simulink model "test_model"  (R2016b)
settings: Solver=VariableStepAuto  StartTime=0.0  StopTime=runtime  RelTol=1e-3
InitFcn:
  | clear mex
  | delete test_model_sfun.mexw64
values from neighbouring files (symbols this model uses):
  delta_T = 4 * [ 0,  0,  2.351e-4 ]    [modelParameters.m]
  Delta_T = cell(1,4)    [modelParameters.m]
  F_D = 1*randn(3,1)    [modelParameters.m]
  g = 9.81    [modelParameters.m]    (also in analyzeIMU_data.m = 9.8; getMomentOfInertia.m = 9.80665)
  Gamma_H = cell(1,4)    [modelParameters.m]
  have_motor_transient = 1    [modelParameters.m]
  height_controlled_o = (((Rm*If        + (((omega0_o * 2 * Rm * Kv * Kq      * Kd + 1)^2) - 1)/(4* Rm*Kv^2*Kq      * Kd))/Vb)*(Pmax - Pmin) + Pmin)    [modelParameters.m]
  i_0 = cell(1,4)    [modelParameters.m]
  If = 0.3836    [modelParameters.m]    (also in thrustDragConstantCalculations.m = [If0; If1; If2; If3]; Kd_error.m = I_0 * sign(rotor_speed_0) + I_1 * rotor_speed_0 + I_2 * roto)
  J = diag([ 0.0130 0.0140 0.0285 ])    [modelParameters.m]    (also in J_calc_bifilar.m = (16*pi^2*L./(m*g.*D.^2))\(t./n).^2)
  J_L = m_L/12*diag([y_L^2+z_L^2,x_L^2+z_L^2,x_L^2+y_L^2])    [modelParameters.m]
  J_r = cell(1,4)    [modelParameters.m]
  Jreq = 4.2012e-05    [modelParameters.m]
  Jxx = 0.0130    (= 0.013)    [modelParameters.m]
  Jyy = 0.0140    (= 0.014)    [modelParameters.m]
  Jzz = 0.0285    [modelParameters.m]
  K_d = cell(1,4)    [modelParameters.m]
  K_E = cell(1,4)    [modelParameters.m]
  K_H = cell(1,4)    [modelParameters.m]
  K_Q = cell(1,4)    [modelParameters.m]
  K_T = cell(1,4)    [modelParameters.m]
  K_V = cell(1,4)    [modelParameters.m]
  Kd = 1.4852e-07    [modelParameters.m]    (also in calcDragConstant.m = ((A'*A)^-1)*A'*b; thrustDragConstantCalculations.m = calcDragConstant(data, Pmin, Pmax, Rm, Kv, Kq, If); Kd_error.m = 1.0317e-07)
  Kh = 3.4574e-04    (= 0.00034574)    [modelParameters.m]
  Ki_mahony = 0.001    [modelParameters.m]
  Kp_mahony = 0.4    [modelParameters.m]
  Kq = 96.3422    [modelParameters.m]    (also in thrustDragConstantCalculations.m; Kd_error.m)
  Kt = 1.2007e-05    [modelParameters.m]    (also in calcThrustConstant.m = ((A'*A)^(-1))*(A'*T); thrustDragConstantCalculations.m = calcThrustConstant(data))
  Kv = 96.3422    [modelParameters.m]    (also in thrustDragConstantCalculations.m; Kd_error.m)
  m = 1.216    [modelParameters.m]
  m_L = 0    [modelParameters.m]
  omega0_o = sqrt((m*g)/(4*Kt))    [modelParameters.m]
  omega1_o = sqrt((m*g)/(4*Kt))    [modelParameters.m]
  omega2_o = sqrt((m*g)/(4*Kt))    [modelParameters.m]
  omega3_o = sqrt((m*g)/(4*Kt))    [modelParameters.m]
  omega_0 = cell(1,4)    [modelParameters.m]
  p0 = 0    [modelParameters.m]
  p_0 = cell(1,4)    [modelParameters.m]
  p_max = cell(1,4)    [modelParameters.m]
  phi0 = 0    [modelParameters.m]
  pitch_o = 0    [modelParameters.m]
  pitchrate_o = 0    [modelParameters.m]
  Pmax = 1    [modelParameters.m]    (also in thrustDragConstantCalculations.m = 200000; Kd_error.m = 200000)
  Pmin = 0    [modelParameters.m]    (also in thrustDragConstantCalculations.m = 100000; Kd_error.m = 100000)
  psi0 = 0    [modelParameters.m]
  q0 = 0    [modelParameters.m]
  Q_D = 0.05*randn(3,1)    [modelParameters.m]
  r0 = 0    [modelParameters.m]
  R_m = cell(1,4)    [modelParameters.m]
  r_oc = [ 0 ; 0 ; 0 ]    [modelParameters.m]
  r_oL = [0; 0; 0]    [modelParameters.m]
  rhx = 0.16    [modelParameters.m]
  rhy = 0.16    [modelParameters.m]
  rhz = 0.03    [modelParameters.m]
  Rm = 0.235    [modelParameters.m]    (also in thrustDragConstantCalculations.m = 0.2308; Kd_error.m = 0.2308)
  roll_o = 0    [modelParameters.m]
  rollrate_o = 0    [modelParameters.m]
  Tc = 0.04    [modelParameters.m]
  theta0 = 0    [modelParameters.m]
  Tq = 0.005    [modelParameters.m]
  u0 = 0    [modelParameters.m]
  v0 = 0    [modelParameters.m]
  Vb = 12.3    [modelParameters.m]    (also in calcDragConstant.m = [data.(6); data.(6); data.(6); data.(6)]; Kd_error.m = data.(6))
  w0 = 0    [modelParameters.m]
  x0 = 0    [modelParameters.m]
  x_controlled_o = 0    [modelParameters.m]
  x_o = 0    [modelParameters.m]
  x_vel_o = 0    [modelParameters.m]
  y0 = 0    [modelParameters.m]
  y_controlled_o = 0    [modelParameters.m]
  y_o = 0    [modelParameters.m]
  y_vel_o = 0    [modelParameters.m]
  yaw_controlled_o = 0    [modelParameters.m]
  yaw_o = 0    [modelParameters.m]
  yawrate_o = 0    [modelParameters.m]
  z0 = 0    [modelParameters.m]
  z_o = 0    [modelParameters.m]
  z_vel_o = 0    [modelParameters.m]
undefined symbols (not defined in the file or in its folder): Gamma_Omega, Gamma_T, Ki, Kp, r_h, slope, start, Ts, X0
libraries: simulink x32, Derivative x26, dsparch4 x6, vrlib x4
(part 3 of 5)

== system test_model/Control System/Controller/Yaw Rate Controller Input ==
  note: 1) Add Subsystem or Model blocks as valid variant choices. 2) You cannot connect blocks at this level. At simulation, connectivity is automatically determined, based on the active variant and port name matching.
  yawrate_error_model : Inport
  yawrate_model : Inport  Port=2
  Feedback : Subsystem  VariantControl=logAnalysisToggle==0
  yawrate error : Subsystem  VariantControl=logAnalysisToggle==1
  yawrate_error : Outport
  yawrate : Outport  Port=2

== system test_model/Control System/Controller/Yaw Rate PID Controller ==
  yawrate_error : Inport
  yawrate : Inport  Port=2
  Add : Sum  Inputs=+-
  Discrete D Controller : Derivative/Discrete D Controller  Kd=Kd  a=a
  Discrete PI Controller : simulink/Continuous/PID Controller  Controller=PI  TimeDomain=Discrete-time  SampleTime=Ts  IntegratorMethod=Forward Euler  FilterMethod=Forward Euler  Form=Parallel  UseFilter=on  ControllerParametersSource=internal  P=Kp  I=Ki  D=0  N=100  InitialConditionSource=internal  InitialConditionForIntegrator=0  InitialConditionForFilter=0  ExternalReset=none  LimitOutput=off  UpperSaturationLimit=inf  LowerSaturationLimit=-inf  LinearizeAsGain=off  AntiWindupMode=none  Kb=1  TrackingMode=off  Kt=1  PParamMin=[]  PParamMax=[]  IParamMin=[]  IParamMax=[]  DParamMin=[]  DParamMax=[]  NParamMin=[]  NParamMax=[]  KbParamMin=[]  KbParamMax=[]  KtParamMin=[]  KtParamMax=[]  POutMin=[]  POutMax=[]  IOutMin=[]  IOutMax=[]  DOutMin=[]  DOutMax=[]  NOutMin=[]  NOutMax=[]  KbOutMin=[]  KbOutMax=[]  KtOutMin=[]  KtOutMax=[]  IntegratorOutMin=[]  IntegratorOutMax=[]  FilterOutMin=[]  FilterOutMax=[]  SumOutMin=[]  SumOutMax=[]  SumI1OutMin=[]  SumI1OutMax=[]  SumI2OutMin=[]  SumI2OutMax=[]  SumI3OutMin=[]  SumI3OutMax=[]  SumDOutMin=[]  SumDOutMax=[]  SaturationOutMin=[]  SaturationOutMax=[]  IntegratorContinuousStateAttributes=''  IntegratorStateMustResolveToSignalObject=off  IntegratorRTWStateStorageClass=Auto  FilterContinuousStateAttributes=''  FilterStateMustResolveToSignalObject=off  FilterRTWStateStorageClass=Auto  DifferentiatorICPrevScaledInput=0  DifferentiatorOutMin=[]  DifferentiatorOutMax=[]
  yaw_motor_command : Outport
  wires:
  yawrate/1 -> Discrete D Controller/1
  yawrate_error/1 -> Discrete PI Controller/1
  Discrete PI Controller/1 -> Add/1
  Discrete D Controller/1 -> Add/2
  Add/1 -> yaw_motor_command/1

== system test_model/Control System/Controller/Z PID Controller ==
  z_error : Inport
  z_pos : Inport  Port=2
  Add : Sum  Inputs=+-
  Discrete D Controller : Derivative/Discrete D Controller  Kd=Kd  a=a
  Discrete PI Controller : simulink/Continuous/PID Controller  Controller=PI  TimeDomain=Discrete-time  SampleTime=Ts  IntegratorMethod=Forward Euler  FilterMethod=Forward Euler  Form=Parallel  UseFilter=on  ControllerParametersSource=internal  P=Kp  I=Ki  D=0  N=100  InitialConditionSource=internal  InitialConditionForIntegrator=0  InitialConditionForFilter=0  ExternalReset=none  LimitOutput=off  UpperSaturationLimit=inf  LowerSaturationLimit=-inf  LinearizeAsGain=off  AntiWindupMode=none  Kb=1  TrackingMode=off  Kt=1  PParamMin=[]  PParamMax=[]  IParamMin=[]  IParamMax=[]  DParamMin=[]  DParamMax=[]  NParamMin=[]  NParamMax=[]  KbParamMin=[]  KbParamMax=[]  KtParamMin=[]  KtParamMax=[]  POutMin=[]  POutMax=[]  IOutMin=[]  IOutMax=[]  DOutMin=[]  DOutMax=[]  NOutMin=[]  NOutMax=[]  KbOutMin=[]  KbOutMax=[]  KtOutMin=[]  KtOutMax=[]  IntegratorOutMin=[]  IntegratorOutMax=[]  FilterOutMin=[]  FilterOutMax=[]  SumOutMin=[]  SumOutMax=[]  SumI1OutMin=[]  SumI1OutMax=[]  SumI2OutMin=[]  SumI2OutMax=[]  SumI3OutMin=[]  SumI3OutMax=[]  SumDOutMin=[]  SumDOutMax=[]  SaturationOutMin=[]  SaturationOutMax=[]  IntegratorContinuousStateAttributes=''  IntegratorStateMustResolveToSignalObject=off  IntegratorRTWStateStorageClass=Auto  FilterContinuousStateAttributes=''  FilterStateMustResolveToSignalObject=off  FilterRTWStateStorageClass=Auto  DifferentiatorICPrevScaledInput=0  DifferentiatorOutMin=[]  DifferentiatorOutMax=[]
  z_motor_command : Outport
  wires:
  z_pos/1 -> Discrete D Controller/1
  z_error/1 -> Discrete PI Controller/1
  Discrete PI Controller/1 -> Add/1
  Discrete D Controller/1 -> Add/2
  Add/1 -> z_motor_command/1

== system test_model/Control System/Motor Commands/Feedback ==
  z_command_model : Inport
  z_command : Outport
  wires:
  z_command_model/1 -> z_command/1

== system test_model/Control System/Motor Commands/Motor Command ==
  From Workspace5 : FromWorkspace  VariableName=motor_commands  SampleTime=Tq
  z_command : Outport
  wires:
  From Workspace5/1 -> z_command/1

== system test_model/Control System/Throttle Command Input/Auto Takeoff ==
  height_controlled_o : Constant  Value=0.45  SampleTime=Tc
  z_command : Outport
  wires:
  height_controlled_o/1 -> z_command/1

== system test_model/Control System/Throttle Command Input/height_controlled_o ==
  height_controlled_o : Constant  Value=height_controlled_o  SampleTime=Tc
  z_command : Outport
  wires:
  height_controlled_o/1 -> z_command/1

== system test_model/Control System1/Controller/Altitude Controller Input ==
  note: 1) Add Subsystem or Model blocks as valid variant choices. 2) You cannot connect blocks at this level. At simulation, connectivity is automatically determined, based on the active variant and port name matching.
  z_error_model : Inport
  z_position_model : Inport  Port=2
  Feedback : Subsystem  VariantControl=logAnalysisToggle==0
  z error : Subsystem  VariantControl=logAnalysisToggle==1
  z_error : Outport
  z_position : Outport  Port=2

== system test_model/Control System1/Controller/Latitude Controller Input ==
  note: 1) Add Subsystem or Model blocks as valid variant choices. 2) You cannot connect blocks at this level. At simulation, connectivity is automatically determined, based on the active variant and port name matching.
  x_error_model : Inport
  x_position_model : Inport  Port=2
  Feedback : Subsystem  VariantControl=logAnalysisToggle==0
  log : Subsystem  VariantControl=logAnalysisToggle==1
  x_error : Outport
  x_position : Outport  Port=2

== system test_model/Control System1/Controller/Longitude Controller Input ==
  note: 1) Add Subsystem or Model blocks as valid variant choices. 2) You cannot connect blocks at this level. At simulation, connectivity is automatically determined, based on the active variant and port name matching.
  y_error_model : Inport
  y_position_model : Inport  Port=2
  Feedback : Subsystem  VariantControl=logAnalysisToggle==0
  y error : Subsystem  VariantControl=logAnalysisToggle==1
  y_error : Outport
  y_position : Outport  Port=2

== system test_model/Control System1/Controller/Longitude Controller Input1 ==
  note: 1) Add Subsystem or Model blocks as valid variant choices. 2) You cannot connect blocks at this level. At simulation, connectivity is automatically determined, based on the active variant and port name matching.
  y_vel_error_model : Inport
  y_vel_model : Inport  Port=2
  Feedback : Subsystem  VariantControl=logAnalysisToggle==0
  y error : Subsystem  VariantControl=logAnalysisToggle==1
  y_vel_error : Outport
  y_vel : Outport  Port=2

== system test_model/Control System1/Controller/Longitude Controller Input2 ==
  note: 1) Add Subsystem or Model blocks as valid variant choices. 2) You cannot connect blocks at this level. At simulation, connectivity is automatically determined, based on the active variant and port name matching.
  x_vel_error_model : Inport
  x_vel_model : Inport  Port=2
  Feedback : Subsystem  VariantControl=logAnalysisToggle==0
  y error : Subsystem  VariantControl=logAnalysisToggle==1
  x_vel_error : Outport
  x_vel : Outport  Port=2

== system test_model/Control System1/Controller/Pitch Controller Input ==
  note: 1) Add Subsystem or Model blocks as valid variant choices. 2) You cannot connect blocks at this level. At simulation, connectivity is automatically determined, based on the active variant and port name matching.
  pitch_error_model : Inport
  pitch_angle_model : Inport  Port=2
  Feedback : Subsystem  VariantControl=logAnalysisToggle==0
  pitch error : Subsystem  VariantControl=logAnalysisToggle==1
  pitch_error : Outport
  pitch_angle : Outport  Port=2

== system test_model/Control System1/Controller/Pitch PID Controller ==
  pitch_error : Inport
  pitch_angle : Inport  Port=2
  Add : Sum  Inputs=+-
  Discrete D Controller : Derivative/Discrete D Controller  Kd=Kd  a=a
  Discrete PI Controller : simulink/Continuous/PID Controller  Controller=PI  TimeDomain=Discrete-time  SampleTime=Ts  IntegratorMethod=Forward Euler  FilterMethod=Forward Euler  Form=Parallel  UseFilter=on  ControllerParametersSource=internal  P=Kp  I=Ki  D=0  N=100  InitialConditionSource=internal  InitialConditionForIntegrator=0  InitialConditionForFilter=0  ExternalReset=none  LimitOutput=off  UpperSaturationLimit=inf  LowerSaturationLimit=-inf  LinearizeAsGain=off  AntiWindupMode=none  Kb=1  TrackingMode=off  Kt=1  PParamMin=[]  PParamMax=[]  IParamMin=[]  IParamMax=[]  DParamMin=[]  DParamMax=[]  NParamMin=[]  NParamMax=[]  KbParamMin=[]  KbParamMax=[]  KtParamMin=[]  KtParamMax=[]  POutMin=[]  POutMax=[]  IOutMin=[]  IOutMax=[]  DOutMin=[]  DOutMax=[]  NOutMin=[]  NOutMax=[]  KbOutMin=[]  KbOutMax=[]  KtOutMin=[]  KtOutMax=[]  IntegratorOutMin=[]  IntegratorOutMax=[]  FilterOutMin=[]  FilterOutMax=[]  SumOutMin=[]  SumOutMax=[]  SumI1OutMin=[]  SumI1OutMax=[]  SumI2OutMin=[]  SumI2OutMax=[]  SumI3OutMin=[]  SumI3OutMax=[]  SumDOutMin=[]  SumDOutMax=[]  SaturationOutMin=[]  SaturationOutMax=[]  IntegratorContinuousStateAttributes=''  IntegratorStateMustResolveToSignalObject=off  IntegratorRTWStateStorageClass=Auto  FilterContinuousStateAttributes=''  FilterStateMustResolveToSignalObject=off  FilterRTWStateStorageClass=Auto  DifferentiatorICPrevScaledInput=0  DifferentiatorOutMin=[]  DifferentiatorOutMax=[]
  pitchrate_setpoint : Outport
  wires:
  pitch_angle/1 -> Discrete D Controller/1
  pitch_error/1 -> Discrete PI Controller/1
  Discrete PI Controller/1 -> Add/1
  Discrete D Controller/1 -> Add/2
  Add/1 -> pitchrate_setpoint/1

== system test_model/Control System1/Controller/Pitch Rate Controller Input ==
  note: 1) Add Subsystem or Model blocks as valid variant choices. 2) You cannot connect blocks at this level. At simulation, connectivity is automatically determined, based on the active variant and port name matching.
  pitchrate_error_model : Inport
  pitchrate_model : Inport  Port=2
  Feedback : Subsystem  VariantControl=logAnalysisToggle==0
  pitchrate error : Subsystem  VariantControl=logAnalysisToggle==1
  pitchrate_error : Outport
  pitchrate : Outport  Port=2

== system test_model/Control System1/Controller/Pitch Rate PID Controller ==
  pitchrate_error : Inport
  pitchrate : Inport  Port=2
  Add : Sum  Inputs=+-
  Discrete D Controller : Derivative/Discrete D Controller  Kd=Kd  a=a
  Discrete PI Controller : simulink/Continuous/PID Controller  Controller=PI  TimeDomain=Discrete-time  SampleTime=Ts  IntegratorMethod=Forward Euler  FilterMethod=Forward Euler  Form=Parallel  UseFilter=on  ControllerParametersSource=internal  P=Kp  I=Ki  D=0  N=100  InitialConditionSource=internal  InitialConditionForIntegrator=0  InitialConditionForFilter=0  ExternalReset=none  LimitOutput=off  UpperSaturationLimit=inf  LowerSaturationLimit=-inf  LinearizeAsGain=off  AntiWindupMode=none  Kb=1  TrackingMode=off  Kt=1  PParamMin=[]  PParamMax=[]  IParamMin=[]  IParamMax=[]  DParamMin=[]  DParamMax=[]  NParamMin=[]  NParamMax=[]  KbParamMin=[]  KbParamMax=[]  KtParamMin=[]  KtParamMax=[]  POutMin=[]  POutMax=[]  IOutMin=[]  IOutMax=[]  DOutMin=[]  DOutMax=[]  NOutMin=[]  NOutMax=[]  KbOutMin=[]  KbOutMax=[]  KtOutMin=[]  KtOutMax=[]  IntegratorOutMin=[]  IntegratorOutMax=[]  FilterOutMin=[]  FilterOutMax=[]  SumOutMin=[]  SumOutMax=[]  SumI1OutMin=[]  SumI1OutMax=[]  SumI2OutMin=[]  SumI2OutMax=[]  SumI3OutMin=[]  SumI3OutMax=[]  SumDOutMin=[]  SumDOutMax=[]  SaturationOutMin=[]  SaturationOutMax=[]  IntegratorContinuousStateAttributes=''  IntegratorStateMustResolveToSignalObject=off  IntegratorRTWStateStorageClass=Auto  FilterContinuousStateAttributes=''  FilterStateMustResolveToSignalObject=off  FilterRTWStateStorageClass=Auto  DifferentiatorICPrevScaledInput=0  DifferentiatorOutMin=[]  DifferentiatorOutMax=[]
  x_motor_command : Outport
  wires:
  pitchrate/1 -> Discrete D Controller/1
  pitchrate_error/1 -> Discrete PI Controller/1
  Discrete PI Controller/1 -> Add/1
  Discrete D Controller/1 -> Add/2
  Add/1 -> x_motor_command/1

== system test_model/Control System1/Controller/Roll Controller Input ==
  note: 1) Add Subsystem or Model blocks as valid variant choices. 2) You cannot connect blocks at this level. At simulation, connectivity is automatically determined, based on the active variant and port name matching.
  roll_error_model : Inport
  roll_angle_model : Inport  Port=2
  Feedback : Subsystem  VariantControl=logAnalysisToggle==0
  roll error : Subsystem  VariantControl=logAnalysisToggle==1
  roll_error : Outport
  roll_angle : Outport  Port=2

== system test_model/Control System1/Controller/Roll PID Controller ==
  roll_error : Inport
  roll_angle : Inport  Port=2
  Add : Sum  Inputs=+-
  Discrete D Controller : Derivative/Discrete D Controller  Kd=Kd  a=a
  Discrete PI Controller : simulink/Continuous/PID Controller  Controller=PI  TimeDomain=Discrete-time  SampleTime=Ts  IntegratorMethod=Forward Euler  FilterMethod=Forward Euler  Form=Parallel  UseFilter=on  ControllerParametersSource=internal  P=Kp  I=Ki  D=0  N=100  InitialConditionSource=internal  InitialConditionForIntegrator=0  InitialConditionForFilter=0  ExternalReset=none  LimitOutput=off  UpperSaturationLimit=inf  LowerSaturationLimit=-inf  LinearizeAsGain=off  AntiWindupMode=none  Kb=1  TrackingMode=off  Kt=1  PParamMin=[]  PParamMax=[]  IParamMin=[]  IParamMax=[]  DParamMin=[]  DParamMax=[]  NParamMin=[]  NParamMax=[]  KbParamMin=[]  KbParamMax=[]  KtParamMin=[]  KtParamMax=[]  POutMin=[]  POutMax=[]  IOutMin=[]  IOutMax=[]  DOutMin=[]  DOutMax=[]  NOutMin=[]  NOutMax=[]  KbOutMin=[]  KbOutMax=[]  KtOutMin=[]  KtOutMax=[]  IntegratorOutMin=[]  IntegratorOutMax=[]  FilterOutMin=[]  FilterOutMax=[]  SumOutMin=[]  SumOutMax=[]  SumI1OutMin=[]  SumI1OutMax=[]  SumI2OutMin=[]  SumI2OutMax=[]  SumI3OutMin=[]  SumI3OutMax=[]  SumDOutMin=[]  SumDOutMax=[]  SaturationOutMin=[]  SaturationOutMax=[]  IntegratorContinuousStateAttributes=''  IntegratorStateMustResolveToSignalObject=off  IntegratorRTWStateStorageClass=Auto  FilterContinuousStateAttributes=''  FilterStateMustResolveToSignalObject=off  FilterRTWStateStorageClass=Auto  DifferentiatorICPrevScaledInput=0  DifferentiatorOutMin=[]  DifferentiatorOutMax=[]
  rollrate_setpoint : Outport
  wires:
  roll_angle/1 -> Discrete D Controller/1
  roll_error/1 -> Discrete PI Controller/1
  Discrete PI Controller/1 -> Add/1
  Discrete D Controller/1 -> Add/2
  Add/1 -> rollrate_setpoint/1

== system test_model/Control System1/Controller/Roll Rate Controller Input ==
  note: 1) Add Subsystem or Model blocks as valid variant choices. 2) You cannot connect blocks at this level. At simulation, connectivity is automatically determined, based on the active variant and port name matching.
  rollrate_error_model : Inport
  rollrate_model : Inport  Port=2
  Feedback : Subsystem  VariantControl=logAnalysisToggle==0
  rollrate error : Subsystem  VariantControl=logAnalysisToggle==1
  rollrate_error : Outport
  rollrate : Outport  Port=2

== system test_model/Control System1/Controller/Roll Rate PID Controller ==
  rollrate_error : Inport
  rollrate : Inport  Port=2
  Add : Sum  Inputs=+-
  Discrete D Controller : Derivative/Discrete D Controller  Kd=Kd  a=a
  Discrete PI Controller : simulink/Continuous/PID Controller  Controller=PI  TimeDomain=Discrete-time  SampleTime=Ts  IntegratorMethod=Forward Euler  FilterMethod=Forward Euler  Form=Parallel  UseFilter=on  ControllerParametersSource=internal  P=Kp  I=Ki  D=0  N=100  InitialConditionSource=internal  InitialConditionForIntegrator=0  InitialConditionForFilter=0  ExternalReset=none  LimitOutput=off  UpperSaturationLimit=inf  LowerSaturationLimit=-inf  LinearizeAsGain=off  AntiWindupMode=none  Kb=1  TrackingMode=off  Kt=1  PParamMin=[]  PParamMax=[]  IParamMin=[]  IParamMax=[]  DParamMin=[]  DParamMax=[]  NParamMin=[]  NParamMax=[]  KbParamMin=[]  KbParamMax=[]  KtParamMin=[]  KtParamMax=[]  POutMin=[]  POutMax=[]  IOutMin=[]  IOutMax=[]  DOutMin=[]  DOutMax=[]  NOutMin=[]  NOutMax=[]  KbOutMin=[]  KbOutMax=[]  KtOutMin=[]  KtOutMax=[]  IntegratorOutMin=[]  IntegratorOutMax=[]  FilterOutMin=[]  FilterOutMax=[]  SumOutMin=[]  SumOutMax=[]  SumI1OutMin=[]  SumI1OutMax=[]  SumI2OutMin=[]  SumI2OutMax=[]  SumI3OutMin=[]  SumI3OutMax=[]  SumDOutMin=[]  SumDOutMax=[]  SaturationOutMin=[]  SaturationOutMax=[]  IntegratorContinuousStateAttributes=''  IntegratorStateMustResolveToSignalObject=off  IntegratorRTWStateStorageClass=Auto  FilterContinuousStateAttributes=''  FilterStateMustResolveToSignalObject=off  FilterRTWStateStorageClass=Auto  DifferentiatorICPrevScaledInput=0  DifferentiatorOutMin=[]  DifferentiatorOutMax=[]
  y_motor_command : Outport
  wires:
  rollrate/1 -> Discrete D Controller/1
  rollrate_error/1 -> Discrete PI Controller/1
  Discrete PI Controller/1 -> Add/1
  Discrete D Controller/1 -> Add/2
  Add/1 -> y_motor_command/1

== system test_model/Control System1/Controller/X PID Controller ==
  x_error : Inport
  x_pos : Inport  Port=2
  Add : Sum  Inputs=+-
  Discrete D Controller : Derivative/Discrete D Controller  Kd=Kd  a=a
  Discrete PI Controller : simulink/Continuous/PID Controller  Controller=PI  TimeDomain=Discrete-time  SampleTime=Ts  IntegratorMethod=Forward Euler  FilterMethod=Forward Euler  Form=Parallel  UseFilter=on  ControllerParametersSource=internal  P=Kp  I=Ki  D=0  N=100  InitialConditionSource=internal  InitialConditionForIntegrator=0  InitialConditionForFilter=0  ExternalReset=none  LimitOutput=off  UpperSaturationLimit=inf  LowerSaturationLimit=-inf  LinearizeAsGain=off  AntiWindupMode=none  Kb=1  TrackingMode=off  Kt=1  PParamMin=[]  PParamMax=[]  IParamMin=[]  IParamMax=[]  DParamMin=[]  DParamMax=[]  NParamMin=[]  NParamMax=[]  KbParamMin=[]  KbParamMax=[]  KtParamMin=[]  KtParamMax=[]  POutMin=[]  POutMax=[]  IOutMin=[]  IOutMax=[]  DOutMin=[]  DOutMax=[]  NOutMin=[]  NOutMax=[]  KbOutMin=[]  KbOutMax=[]  KtOutMin=[]  KtOutMax=[]  IntegratorOutMin=[]  IntegratorOutMax=[]  FilterOutMin=[]  FilterOutMax=[]  SumOutMin=[]  SumOutMax=[]  SumI1OutMin=[]  SumI1OutMax=[]  SumI2OutMin=[]  SumI2OutMax=[]  SumI3OutMin=[]  SumI3OutMax=[]  SumDOutMin=[]  SumDOutMax=[]  SaturationOutMin=[]  SaturationOutMax=[]  IntegratorContinuousStateAttributes=''  IntegratorStateMustResolveToSignalObject=off  IntegratorRTWStateStorageClass=Auto  FilterContinuousStateAttributes=''  FilterStateMustResolveToSignalObject=off  FilterRTWStateStorageClass=Auto  DifferentiatorICPrevScaledInput=0  DifferentiatorOutMin=[]  DifferentiatorOutMax=[]
  pitch_setpoint : Outport
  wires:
  x_pos/1 -> Discrete D Controller/1
  x_error/1 -> Discrete PI Controller/1
  Discrete PI Controller/1 -> Add/1
  Discrete D Controller/1 -> Add/2
  Add/1 -> pitch_setpoint/1

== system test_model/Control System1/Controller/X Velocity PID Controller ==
  x_vel_error : Inport
  x_vel : Inport  Port=2
  Add : Sum  Inputs=+-
  Discrete D Controller : Derivative/Discrete D Controller  Kd=Kd  a=a
  Discrete PI Controller : simulink/Continuous/PID Controller  Controller=PI  TimeDomain=Discrete-time  SampleTime=Ts  IntegratorMethod=Forward Euler  FilterMethod=Forward Euler  Form=Parallel  UseFilter=on  ControllerParametersSource=internal  P=Kp  I=Ki  D=0  N=100  InitialConditionSource=internal  InitialConditionForIntegrator=0  InitialConditionForFilter=0  ExternalReset=none  LimitOutput=off  UpperSaturationLimit=inf  LowerSaturationLimit=-inf  LinearizeAsGain=off  AntiWindupMode=none  Kb=1  TrackingMode=off  Kt=1  PParamMin=[]  PParamMax=[]  IParamMin=[]  IParamMax=[]  DParamMin=[]  DParamMax=[]  NParamMin=[]  NParamMax=[]  KbParamMin=[]  KbParamMax=[]  KtParamMin=[]  KtParamMax=[]  POutMin=[]  POutMax=[]  IOutMin=[]  IOutMax=[]  DOutMin=[]  DOutMax=[]  NOutMin=[]  NOutMax=[]  KbOutMin=[]  KbOutMax=[]  KtOutMin=[]  KtOutMax=[]  IntegratorOutMin=[]  IntegratorOutMax=[]  FilterOutMin=[]  FilterOutMax=[]  SumOutMin=[]  SumOutMax=[]  SumI1OutMin=[]  SumI1OutMax=[]  SumI2OutMin=[]  SumI2OutMax=[]  SumI3OutMin=[]  SumI3OutMax=[]  SumDOutMin=[]  SumDOutMax=[]  SaturationOutMin=[]  SaturationOutMax=[]  IntegratorContinuousStateAttributes=''  IntegratorStateMustResolveToSignalObject=off  IntegratorRTWStateStorageClass=Auto  FilterContinuousStateAttributes=''  FilterStateMustResolveToSignalObject=off  FilterRTWStateStorageClass=Auto  DifferentiatorICPrevScaledInput=0  DifferentiatorOutMin=[]  DifferentiatorOutMax=[]
  pitch_setpoint : Outport
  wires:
  x_vel/1 -> Discrete D Controller/1
  x_vel_error/1 -> Discrete PI Controller/1
  Discrete PI Controller/1 -> Add/1
  Discrete D Controller/1 -> Add/2
  Add/1 -> pitch_setpoint/1

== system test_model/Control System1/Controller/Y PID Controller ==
  y_error : Inport
  y_pos : Inport  Port=2
  Add : Sum  Inputs=+-
  Discrete D Controller : Derivative/Discrete D Controller  Kd=Kd  a=a
  Discrete PI Controller : simulink/Continuous/PID Controller  Controller=PI  TimeDomain=Discrete-time  SampleTime=Ts  IntegratorMethod=Forward Euler  FilterMethod=Forward Euler  Form=Parallel  UseFilter=on  ControllerParametersSource=internal  P=Kp  I=Ki  D=0  N=100  InitialConditionSource=internal  InitialConditionForIntegrator=0  InitialConditionForFilter=0  ExternalReset=none  LimitOutput=off  UpperSaturationLimit=inf  LowerSaturationLimit=-inf  LinearizeAsGain=off  AntiWindupMode=none  Kb=1  TrackingMode=off  Kt=1  PParamMin=[]  PParamMax=[]  IParamMin=[]  IParamMax=[]  DParamMin=[]  DParamMax=[]  NParamMin=[]  NParamMax=[]  KbParamMin=[]  KbParamMax=[]  KtParamMin=[]  KtParamMax=[]  POutMin=[]  POutMax=[]  IOutMin=[]  IOutMax=[]  DOutMin=[]  DOutMax=[]  NOutMin=[]  NOutMax=[]  KbOutMin=[]  KbOutMax=[]  KtOutMin=[]  KtOutMax=[]  IntegratorOutMin=[]  IntegratorOutMax=[]  FilterOutMin=[]  FilterOutMax=[]  SumOutMin=[]  SumOutMax=[]  SumI1OutMin=[]  SumI1OutMax=[]  SumI2OutMin=[]  SumI2OutMax=[]  SumI3OutMin=[]  SumI3OutMax=[]  SumDOutMin=[]  SumDOutMax=[]  SaturationOutMin=[]  SaturationOutMax=[]  IntegratorContinuousStateAttributes=''  IntegratorStateMustResolveToSignalObject=off  IntegratorRTWStateStorageClass=Auto  FilterContinuousStateAttributes=''  FilterStateMustResolveToSignalObject=off  FilterRTWStateStorageClass=Auto  DifferentiatorICPrevScaledInput=0  DifferentiatorOutMin=[]  DifferentiatorOutMax=[]
  roll_setpoint : Outport
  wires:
  y_pos/1 -> Discrete D Controller/1
  y_error/1 -> Discrete PI Controller/1
  Discrete PI Controller/1 -> Add/1
  Discrete D Controller/1 -> Add/2
  Add/1 -> roll_setpoint/1

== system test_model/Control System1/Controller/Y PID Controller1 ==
  y_error : Inport
  y_pos : Inport  Port=2
  Add : Sum  Inputs=+-
  Discrete D Controller : Derivative/Discrete D Controller  Kd=Kd  a=a
  Discrete PI Controller : simulink/Continuous/PID Controller  Controller=PI  TimeDomain=Discrete-time  SampleTime=Ts  IntegratorMethod=Forward Euler  FilterMethod=Forward Euler  Form=Parallel  UseFilter=on  ControllerParametersSource=internal  P=Kp  I=Ki  D=0  N=100  InitialConditionSource=internal  InitialConditionForIntegrator=0  InitialConditionForFilter=0  ExternalReset=none  LimitOutput=off  UpperSaturationLimit=inf  LowerSaturationLimit=-inf  LinearizeAsGain=off  AntiWindupMode=none  Kb=1  TrackingMode=off  Kt=1  PParamMin=[]  PParamMax=[]  IParamMin=[]  IParamMax=[]  DParamMin=[]  DParamMax=[]  NParamMin=[]  NParamMax=[]  KbParamMin=[]  KbParamMax=[]  KtParamMin=[]  KtParamMax=[]  POutMin=[]  POutMax=[]  IOutMin=[]  IOutMax=[]  DOutMin=[]  DOutMax=[]  NOutMin=[]  NOutMax=[]  KbOutMin=[]  KbOutMax=[]  KtOutMin=[]  KtOutMax=[]  IntegratorOutMin=[]  IntegratorOutMax=[]  FilterOutMin=[]  FilterOutMax=[]  SumOutMin=[]  SumOutMax=[]  SumI1OutMin=[]  SumI1OutMax=[]  SumI2OutMin=[]  SumI2OutMax=[]  SumI3OutMin=[]  SumI3OutMax=[]  SumDOutMin=[]  SumDOutMax=[]  SaturationOutMin=[]  SaturationOutMax=[]  IntegratorContinuousStateAttributes=''  IntegratorStateMustResolveToSignalObject=off  IntegratorRTWStateStorageClass=Auto  FilterContinuousStateAttributes=''  FilterStateMustResolveToSignalObject=off  FilterRTWStateStorageClass=Auto  DifferentiatorICPrevScaledInput=0  DifferentiatorOutMin=[]  DifferentiatorOutMax=[]
  y_vel_setpoint : Outport
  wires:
  y_pos/1 -> Discrete D Controller/1
  y_error/1 -> Discrete PI Controller/1
  Discrete PI Controller/1 -> Add/1
  Discrete D Controller/1 -> Add/2
  Add/1 -> y_vel_setpoint/1

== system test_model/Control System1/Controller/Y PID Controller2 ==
  x_error : Inport
  x_pos : Inport  Port=2
  Add : Sum  Inputs=+-
  Discrete D Controller : Derivative/Discrete D Controller  Kd=Kd  a=a
  Discrete PI Controller : simulink/Continuous/PID Controller  Controller=PI  TimeDomain=Discrete-time  SampleTime=Ts  IntegratorMethod=Forward Euler  FilterMethod=Forward Euler  Form=Parallel  UseFilter=on  ControllerParametersSource=internal  P=Kp  I=Ki  D=0  N=100  InitialConditionSource=internal  InitialConditionForIntegrator=0  InitialConditionForFilter=0  ExternalReset=none  LimitOutput=off  UpperSaturationLimit=inf  LowerSaturationLimit=-inf  LinearizeAsGain=off  AntiWindupMode=none  Kb=1  TrackingMode=off  Kt=1  PParamMin=[]  PParamMax=[]  IParamMin=[]  IParamMax=[]  DParamMin=[]  DParamMax=[]  NParamMin=[]  NParamMax=[]  KbParamMin=[]  KbParamMax=[]  KtParamMin=[]  KtParamMax=[]  POutMin=[]  POutMax=[]  IOutMin=[]  IOutMax=[]  DOutMin=[]  DOutMax=[]  NOutMin=[]  NOutMax=[]  KbOutMin=[]  KbOutMax=[]  KtOutMin=[]  KtOutMax=[]  IntegratorOutMin=[]  IntegratorOutMax=[]  FilterOutMin=[]  FilterOutMax=[]  SumOutMin=[]  SumOutMax=[]  SumI1OutMin=[]  SumI1OutMax=[]  SumI2OutMin=[]  SumI2OutMax=[]  SumI3OutMin=[]  SumI3OutMax=[]  SumDOutMin=[]  SumDOutMax=[]  SaturationOutMin=[]  SaturationOutMax=[]  IntegratorContinuousStateAttributes=''  IntegratorStateMustResolveToSignalObject=off  IntegratorRTWStateStorageClass=Auto  FilterContinuousStateAttributes=''  FilterStateMustResolveToSignalObject=off  FilterRTWStateStorageClass=Auto  DifferentiatorICPrevScaledInput=0  DifferentiatorOutMin=[]  DifferentiatorOutMax=[]
  x_vel_setpoint : Outport
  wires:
  x_pos/1 -> Discrete D Controller/1
  x_error/1 -> Discrete PI Controller/1
  Discrete PI Controller/1 -> Add/1
  Discrete D Controller/1 -> Add/2
  Add/1 -> x_vel_setpoint/1

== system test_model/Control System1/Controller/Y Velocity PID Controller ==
  y_error : Inport
  y_pos : Inport  Port=2
  Add : Sum  Inputs=+-
  Discrete D Controller : Derivative/Discrete D Controller  Kd=Kd  a=a
  Discrete PI Controller : simulink/Continuous/PID Controller  Controller=PI  TimeDomain=Discrete-time  SampleTime=Ts  IntegratorMethod=Forward Euler  FilterMethod=Forward Euler  Form=Parallel  UseFilter=on  ControllerParametersSource=internal  P=Kp  I=Ki  D=0  N=100  InitialConditionSource=internal  InitialConditionForIntegrator=0  InitialConditionForFilter=0  ExternalReset=none  LimitOutput=off  UpperSaturationLimit=inf  LowerSaturationLimit=-inf  LinearizeAsGain=off  AntiWindupMode=none  Kb=1  TrackingMode=off  Kt=1  PParamMin=[]  PParamMax=[]  IParamMin=[]  IParamMax=[]  DParamMin=[]  DParamMax=[]  NParamMin=[]  NParamMax=[]  KbParamMin=[]  KbParamMax=[]  KtParamMin=[]  KtParamMax=[]  POutMin=[]  POutMax=[]  IOutMin=[]  IOutMax=[]  DOutMin=[]  DOutMax=[]  NOutMin=[]  NOutMax=[]  KbOutMin=[]  KbOutMax=[]  KtOutMin=[]  KtOutMax=[]  IntegratorOutMin=[]  IntegratorOutMax=[]  FilterOutMin=[]  FilterOutMax=[]  SumOutMin=[]  SumOutMax=[]  SumI1OutMin=[]  SumI1OutMax=[]  SumI2OutMin=[]  SumI2OutMax=[]  SumI3OutMin=[]  SumI3OutMax=[]  SumDOutMin=[]  SumDOutMax=[]  SaturationOutMin=[]  SaturationOutMax=[]  IntegratorContinuousStateAttributes=''  IntegratorStateMustResolveToSignalObject=off  IntegratorRTWStateStorageClass=Auto  FilterContinuousStateAttributes=''  FilterStateMustResolveToSignalObject=off  FilterRTWStateStorageClass=Auto  DifferentiatorICPrevScaledInput=0  DifferentiatorOutMin=[]  DifferentiatorOutMax=[]
  roll_setpoint : Outport
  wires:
  y_pos/1 -> Discrete D Controller/1
  y_error/1 -> Discrete PI Controller/1
  Discrete PI Controller/1 -> Add/1
  Discrete D Controller/1 -> Add/2
  Add/1 -> roll_setpoint/1

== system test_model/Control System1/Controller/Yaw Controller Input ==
  note: 1) Add Subsystem or Model blocks as valid variant choices. 2) You cannot connect blocks at this level. At simulation, connectivity is automatically determined, based on the active variant and port name matching.
  yaw_error_model : Inport
  yaw_angle_model : Inport  Port=2
  Feedback : Subsystem  VariantControl=logAnalysisToggle==0
  yaw error : Subsystem  VariantControl=logAnalysisToggle==1
  yaw_error : Outport
  yaw_angle : Outport  Port=2

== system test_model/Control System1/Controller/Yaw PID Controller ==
  yaw_error : Inport
  yaw_angle : Inport  Port=2
  Add : Sum  Inputs=+-
  Discrete D Controller : Derivative/Discrete D Controller  Kd=Kd  a=a
  Discrete PI Controller : simulink/Continuous/PID Controller  Controller=PI  TimeDomain=Discrete-time  SampleTime=Ts  IntegratorMethod=Forward Euler  FilterMethod=Forward Euler  Form=Parallel  UseFilter=on  ControllerParametersSource=internal  P=Kp  I=Ki  D=0  N=100  InitialConditionSource=internal  InitialConditionForIntegrator=0  InitialConditionForFilter=0  ExternalReset=none  LimitOutput=off  UpperSaturationLimit=inf  LowerSaturationLimit=-inf  LinearizeAsGain=off  AntiWindupMode=none  Kb=1  TrackingMode=off  Kt=1  PParamMin=[]  PParamMax=[]  IParamMin=[]  IParamMax=[]  DParamMin=[]  DParamMax=[]  NParamMin=[]  NParamMax=[]  KbParamMin=[]  KbParamMax=[]  KtParamMin=[]  KtParamMax=[]  POutMin=[]  POutMax=[]  IOutMin=[]  IOutMax=[]  DOutMin=[]  DOutMax=[]  NOutMin=[]  NOutMax=[]  KbOutMin=[]  KbOutMax=[]  KtOutMin=[]  KtOutMax=[]  IntegratorOutMin=[]  IntegratorOutMax=[]  FilterOutMin=[]  FilterOutMax=[]  SumOutMin=[]  SumOutMax=[]  SumI1OutMin=[]  SumI1OutMax=[]  SumI2OutMin=[]  SumI2OutMax=[]  SumI3OutMin=[]  SumI3OutMax=[]  SumDOutMin=[]  SumDOutMax=[]  SaturationOutMin=[]  SaturationOutMax=[]  IntegratorContinuousStateAttributes=''  IntegratorStateMustResolveToSignalObject=off  IntegratorRTWStateStorageClass=Auto  FilterContinuousStateAttributes=''  FilterStateMustResolveToSignalObject=off  FilterRTWStateStorageClass=Auto  DifferentiatorICPrevScaledInput=0  DifferentiatorOutMin=[]  DifferentiatorOutMax=[]
  yawrate_setpoint : Outport
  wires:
  yaw_angle/1 -> Discrete D Controller/1
  yaw_error/1 -> Discrete PI Controller/1
  Discrete PI Controller/1 -> Add/1
  Discrete D Controller/1 -> Add/2
  Add/1 -> yawrate_setpoint/1

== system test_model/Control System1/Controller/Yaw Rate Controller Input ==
  note: 1) Add Subsystem or Model blocks as valid variant choices. 2) You cannot connect blocks at this level. At simulation, connectivity is automatically determined, based on the active variant and port name matching.
  yawrate_error_model : Inport
  yawrate_model : Inport  Port=2
  Feedback : Subsystem  VariantControl=logAnalysisToggle==0
  yawrate error : Subsystem  VariantControl=logAnalysisToggle==1
  yawrate_error : Outport
  yawrate : Outport  Port=2

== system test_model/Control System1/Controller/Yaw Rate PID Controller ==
  yawrate_error : Inport
  yawrate : Inport  Port=2
  Add : Sum  Inputs=+-
  Discrete D Controller : Derivative/Discrete D Controller  Kd=Kd  a=a
  Discrete PI Controller : simulink/Continuous/PID Controller  Controller=PI  TimeDomain=Discrete-time  SampleTime=Ts  IntegratorMethod=Forward Euler  FilterMethod=Forward Euler  Form=Parallel  UseFilter=on  ControllerParametersSource=internal  P=Kp  I=Ki  D=0  N=100  InitialConditionSource=internal  InitialConditionForIntegrator=0  InitialConditionForFilter=0  ExternalReset=none  LimitOutput=off  UpperSaturationLimit=inf  LowerSaturationLimit=-inf  LinearizeAsGain=off  AntiWindupMode=none  Kb=1  TrackingMode=off  Kt=1  PParamMin=[]  PParamMax=[]  IParamMin=[]  IParamMax=[]  DParamMin=[]  DParamMax=[]  NParamMin=[]  NParamMax=[]  KbParamMin=[]  KbParamMax=[]  KtParamMin=[]  KtParamMax=[]  POutMin=[]  POutMax=[]  IOutMin=[]  IOutMax=[]  DOutMin=[]  DOutMax=[]  NOutMin=[]  NOutMax=[]  KbOutMin=[]  KbOutMax=[]  KtOutMin=[]  KtOutMax=[]  IntegratorOutMin=[]  IntegratorOutMax=[]  FilterOutMin=[]  FilterOutMax=[]  SumOutMin=[]  SumOutMax=[]  SumI1OutMin=[]  SumI1OutMax=[]  SumI2OutMin=[]  SumI2OutMax=[]  SumI3OutMin=[]  SumI3OutMax=[]  SumDOutMin=[]  SumDOutMax=[]  SaturationOutMin=[]  SaturationOutMax=[]  IntegratorContinuousStateAttributes=''  IntegratorStateMustResolveToSignalObject=off  IntegratorRTWStateStorageClass=Auto  FilterContinuousStateAttributes=''  FilterStateMustResolveToSignalObject=off  FilterRTWStateStorageClass=Auto  DifferentiatorICPrevScaledInput=0  DifferentiatorOutMin=[]  DifferentiatorOutMax=[]
  yaw_motor_command : Outport
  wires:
  yawrate/1 -> Discrete D Controller/1
  yawrate_error/1 -> Discrete PI Controller/1
  Discrete PI Controller/1 -> Add/1
  Discrete D Controller/1 -> Add/2
  Add/1 -> yaw_motor_command/1

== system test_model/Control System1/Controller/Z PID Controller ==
  z_error : Inport
  z_pos : Inport  Port=2
  Add : Sum  Inputs=+-
  Discrete D Controller : Derivative/Discrete D Controller  Kd=Kd  a=a
  Discrete PI Controller : simulink/Continuous/PID Controller  Controller=PI  TimeDomain=Discrete-time  SampleTime=Ts  IntegratorMethod=Forward Euler  FilterMethod=Forward Euler  Form=Parallel  UseFilter=on  ControllerParametersSource=internal  P=Kp  I=Ki  D=0  N=100  InitialConditionSource=internal  InitialConditionForIntegrator=0  InitialConditionForFilter=0  ExternalReset=none  LimitOutput=off  UpperSaturationLimit=inf  LowerSaturationLimit=-inf  LinearizeAsGain=off  AntiWindupMode=none  Kb=1  TrackingMode=off  Kt=1  PParamMin=[]  PParamMax=[]  IParamMin=[]  IParamMax=[]  DParamMin=[]  DParamMax=[]  NParamMin=[]  NParamMax=[]  KbParamMin=[]  KbParamMax=[]  KtParamMin=[]  KtParamMax=[]  POutMin=[]  POutMax=[]  IOutMin=[]  IOutMax=[]  DOutMin=[]  DOutMax=[]  NOutMin=[]  NOutMax=[]  KbOutMin=[]  KbOutMax=[]  KtOutMin=[]  KtOutMax=[]  IntegratorOutMin=[]  IntegratorOutMax=[]  FilterOutMin=[]  FilterOutMax=[]  SumOutMin=[]  SumOutMax=[]  SumI1OutMin=[]  SumI1OutMax=[]  SumI2OutMin=[]  SumI2OutMax=[]  SumI3OutMin=[]  SumI3OutMax=[]  SumDOutMin=[]  SumDOutMax=[]  SaturationOutMin=[]  SaturationOutMax=[]  IntegratorContinuousStateAttributes=''  IntegratorStateMustResolveToSignalObject=off  IntegratorRTWStateStorageClass=Auto  FilterContinuousStateAttributes=''  FilterStateMustResolveToSignalObject=off  FilterRTWStateStorageClass=Auto  DifferentiatorICPrevScaledInput=0  DifferentiatorOutMin=[]  DifferentiatorOutMax=[]
  z_motor_command : Outport
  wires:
  z_pos/1 -> Discrete D Controller/1
  z_error/1 -> Discrete PI Controller/1
  Discrete PI Controller/1 -> Add/1
  Discrete D Controller/1 -> Add/2
  Add/1 -> z_motor_command/1

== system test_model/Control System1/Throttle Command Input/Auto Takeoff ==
  height_controlled_o : Constant  Value=0.45  SampleTime=Tc
  z_command : Outport
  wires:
  height_controlled_o/1 -> z_command/1

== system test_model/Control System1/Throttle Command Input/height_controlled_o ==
  height_controlled_o : Constant  Value=height_controlled_o  SampleTime=Tc
  z_command : Outport
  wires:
  height_controlled_o/1 -> z_command/1

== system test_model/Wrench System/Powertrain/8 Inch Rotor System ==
  M : Inport
  Lambda : Inport  Port=2
  8 Inch Rotor 1 : Subsystem
  8 Inch Rotor 2 : Subsystem
  8 Inch Rotor 3 : Subsystem
  8 Inch Rotor 4 : Subsystem
  Bus Creator : BusCreator  Inputs=8
  Bus Selector : BusSelector  OutputSignals=signal1.alpha_1,signal1.omega_1
  Bus Selector1 : BusSelector  OutputSignals=signal2.alpha_2,signal2.omega_2
  Bus Selector2 : BusSelector  OutputSignals=signal3.alpha_3,signal3.omega_3
  Bus Selector3 : BusSelector  OutputSignals=signal4.alpha_4,signal4.omega_4
  Bus Selector{4..7} (4 alike) : BusSelector  OutputSignals=v_o,Omega
  W_r : Outport
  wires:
  8 Inch Rotor 4/1(F) -> Bus Creator/7  "F_r_4"
  8 Inch Rotor 3/2(Q) -> Bus Creator/6  "Q_r_3"
  8 Inch Rotor 3/1(F) -> Bus Creator/5  "F_r_3"
  8 Inch Rotor 2/2(Q) -> Bus Creator/4  "Q_r_2"
  8 Inch Rotor 2/1(F) -> Bus Creator/3  "F_r_2"
  8 Inch Rotor 4/2(Q) -> Bus Creator/8  "Q_r_4"
  8 Inch Rotor 1/2(Q) -> Bus Creator/2  "Q_r_1"
  8 Inch Rotor 1/1(F) -> Bus Creator/1  "F_r_1"
  Bus Creator/1 -> W_r/1
  Bus Selector/1 -> 8 Inch Rotor 1/1(alpha)  "<alpha_1>"
  Bus Selector/2 -> 8 Inch Rotor 1/2(omega)  "<omega_1>"
  Bus Selector4/1 -> 8 Inch Rotor 1/3(v)  "<v_o>"
  Bus Selector4/2 -> 8 Inch Rotor 1/4(Omega)  "<Omega>"
  Bus Selector1/1 -> 8 Inch Rotor 2/1(alpha)  "<alpha_2>"
  Bus Selector1/2 -> 8 Inch Rotor 2/2(omega)  "<omega_2>"
  Bus Selector5/1 -> 8 Inch Rotor 2/3(v)  "<v_o>"
  Bus Selector5/2 -> 8 Inch Rotor 2/4(Omega)  "<Omega>"
  Bus Selector2/1 -> 8 Inch Rotor 3/1(alpha)  "<alpha_3>"
  Bus Selector2/2 -> 8 Inch Rotor 3/2(omega)  "<omega_3>"
  Bus Selector7/1 -> 8 Inch Rotor 3/3(v)  "<v_o>"
  Bus Selector7/2 -> 8 Inch Rotor 3/4(Omega)  "<Omega>"
  Bus Selector3/1 -> 8 Inch Rotor 4/1(alpha)  "<alpha_4>"
  Bus Selector3/2 -> 8 Inch Rotor 4/2(omega)  "<omega_4>"
  Bus Selector6/1 -> 8 Inch Rotor 4/3(v)  "<v_o>"
  Bus Selector6/2 -> 8 Inch Rotor 4/4(Omega)  "<Omega>"
  Lambda/1 -> Bus Selector4/1, Bus Selector5/1, Bus Selector7/1, Bus Selector6/1
  M/1 -> Bus Selector/1, Bus Selector1/1, Bus Selector2/1, Bus Selector3/1

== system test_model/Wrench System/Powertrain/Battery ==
  Ramp : Subsystem
  V : Outport
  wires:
  Ramp/1(Out1) -> V/1

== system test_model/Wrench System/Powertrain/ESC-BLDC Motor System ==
  P : Inport
  V_b : Inport  Port=2
  Bus Creator{,1..3} (4 alike) : BusCreator  Inputs=2
  Bus Creator4 : BusCreator  Inputs=4
  Demux : Demux
  ESC and BLDC Motor 1 : Subsystem
  ESC and BLDC Motor 2 : Subsystem
  ESC and BLDC Motor 3 : Subsystem
  ESC and BLDC Motor 4 : Subsystem
  M : Outport
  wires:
  Bus Creator4/1 -> M/1
  V_b/1 -> ESC and BLDC Motor 4/2(V_b), ESC and BLDC Motor 3/2(V_b), ESC and BLDC Motor 2/2(V_b), ESC and BLDC Motor 1/2(V_b)
  ESC and BLDC Motor 1/2(omega) -> Bus Creator/2  "omega_1"
  ESC and BLDC Motor 1/1(alpha) -> Bus Creator/1  "alpha_1"
  ESC and BLDC Motor 2/1(alpha) -> Bus Creator1/1  "alpha_2"
  ESC and BLDC Motor 2/2(omega) -> Bus Creator1/2  "omega_2"
  ESC and BLDC Motor 3/1(alpha) -> Bus Creator2/1  "alpha_3"
  ESC and BLDC Motor 3/2(omega) -> Bus Creator2/2  "omega_3"
  ESC and BLDC Motor 4/1(alpha) -> Bus Creator3/1  "alpha_4"
  ESC and BLDC Motor 4/2(omega) -> Bus Creator3/2  "omega_4"
  Bus Creator/1 -> Bus Creator4/1
  Bus Creator1/1 -> Bus Creator4/2
  Bus Creator3/1 -> Bus Creator4/4
  Bus Creator2/1 -> Bus Creator4/3
  P/1 -> Demux/1
  Demux/1 -> ESC and BLDC Motor 2/1(p)
  Demux/2 -> ESC and BLDC Motor 1/1(p)
  Demux/3 -> ESC and BLDC Motor 3/1(p)
  Demux/4 -> ESC and BLDC Motor 4/1(p)

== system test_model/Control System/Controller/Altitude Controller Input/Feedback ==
  z_error_model : Inport
  z_position_model : Inport  Port=2
  z_error : Outport
  z_position : Outport  Port=2
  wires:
  z_error_model/1 -> z_error/1
  z_position_model/1 -> z_position/1

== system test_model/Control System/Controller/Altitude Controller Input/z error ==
  From Workspace1 : FromWorkspace  VariableName=z_position  SampleTime=Tc  Interpolate=off  OutputAfterFinalValue=Holding final value
  From Workspace6 : FromWorkspace  VariableName=z_error  SampleTime=Tc  Interpolate=off  OutputAfterFinalValue=Holding final value
  z_error : Outport
  z_position : Outport  Port=2
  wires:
  From Workspace6/1 -> z_error/1
  From Workspace1/1 -> z_position/1

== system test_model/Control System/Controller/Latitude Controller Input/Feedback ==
  x_error_model : Inport
  x_position_model : Inport  Port=2
  x_error : Outport
  x_position : Outport  Port=2
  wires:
  x_error_model/1 -> x_error/1
  x_position_model/1 -> x_position/1

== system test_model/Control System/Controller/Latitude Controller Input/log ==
  From Workspace : FromWorkspace  VariableName=x_error  SampleTime=Tc  Interpolate=off  OutputAfterFinalValue=Holding final value
  From Workspace1 : FromWorkspace  VariableName=x_position  SampleTime=Tc  Interpolate=off  OutputAfterFinalValue=Holding final value
  x_error : Outport
  x_position : Outport  Port=2
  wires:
  From Workspace/1 -> x_error/1
  From Workspace1/1 -> x_position/1

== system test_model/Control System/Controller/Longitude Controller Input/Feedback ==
  y_error_model : Inport
  y_position_model : Inport  Port=2
  y_error : Outport
  y_position : Outport  Port=2
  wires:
  y_error_model/1 -> y_error/1
  y_position_model/1 -> y_position/1

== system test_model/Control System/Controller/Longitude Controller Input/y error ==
  From Workspace1 : FromWorkspace  VariableName=y_position  SampleTime=Tc  Interpolate=off  OutputAfterFinalValue=Holding final value
  From Workspace3 : FromWorkspace  VariableName=y_error  SampleTime=Tc  Interpolate=off  OutputAfterFinalValue=Holding final value
  y_error : Outport
  y_position : Outport  Port=2
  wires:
  From Workspace3/1 -> y_error/1
  From Workspace1/1 -> y_position/1

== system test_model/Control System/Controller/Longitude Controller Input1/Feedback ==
  y_vel_error_model : Inport
  y_vel_model : Inport  Port=2
  y_vel_error : Outport
  y_vel : Outport  Port=2
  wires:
  y_vel_error_model/1 -> y_vel_error/1
  y_vel_model/1 -> y_vel/1

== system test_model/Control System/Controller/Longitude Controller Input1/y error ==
  From Workspace1 : FromWorkspace  VariableName=y_vel  SampleTime=Tc  Interpolate=off  OutputAfterFinalValue=Holding final value
  From Workspace3 : FromWorkspace  VariableName=y_vel_error  SampleTime=Tc  Interpolate=off  OutputAfterFinalValue=Holding final value
  y_vel_error : Outport
  y_vel : Outport  Port=2
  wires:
  From Workspace3/1 -> y_vel_error/1
  From Workspace1/1 -> y_vel/1

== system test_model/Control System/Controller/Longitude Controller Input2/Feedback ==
  x_vel_error_model : Inport
  x_vel_model : Inport  Port=2
  x_vel_error : Outport
  x_vel : Outport  Port=2
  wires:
  x_vel_error_model/1 -> x_vel_error/1
  x_vel_model/1 -> x_vel/1

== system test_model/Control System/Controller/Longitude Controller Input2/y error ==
  From Workspace1 : FromWorkspace  VariableName=x_vel  SampleTime=Tc  Interpolate=off  OutputAfterFinalValue=Holding final value
  From Workspace3 : FromWorkspace  VariableName=x_vel_error  SampleTime=Tc  Interpolate=off  OutputAfterFinalValue=Holding final value
  x_vel_error : Outport
  x_vel : Outport  Port=2
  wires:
  From Workspace3/1 -> x_vel_error/1
  From Workspace1/1 -> x_vel/1

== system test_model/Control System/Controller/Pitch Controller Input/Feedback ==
  pitch_error_model : Inport
  pitch_angle_model : Inport  Port=2
  pitch_error : Outport
  pitch_angle : Outport  Port=2
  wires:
  pitch_error_model/1 -> pitch_error/1
  pitch_angle_model/1 -> pitch_angle/1

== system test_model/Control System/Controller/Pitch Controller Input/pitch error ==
  From Workspace : FromWorkspace  VariableName=pitch_error  SampleTime=Tq  Interpolate=off  OutputAfterFinalValue=Holding final value
  From Workspace1 : FromWorkspace  VariableName=pitch_angle  SampleTime=Tq  Interpolate=off  OutputAfterFinalValue=Holding final value
  pitch_error : Outport
  pitch_angle : Outport  Port=2
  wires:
  From Workspace/1 -> pitch_error/1
  From Workspace1/1 -> pitch_angle/1

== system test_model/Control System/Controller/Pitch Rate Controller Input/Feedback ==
  pitchrate_error_model : Inport
  pitchrate_model : Inport  Port=2
  pitchrate_error : Outport
  pitchrate : Outport  Port=2
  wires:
  pitchrate_error_model/1 -> pitchrate_error/1
  pitchrate_model/1 -> pitchrate/1

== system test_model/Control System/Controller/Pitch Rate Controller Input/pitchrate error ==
  From Workspace1 : FromWorkspace  VariableName=pitchrate  SampleTime=Tq  Interpolate=off  OutputAfterFinalValue=Holding final value
  From Workspace2 : FromWorkspace  VariableName=pitchrate_error  SampleTime=Tq  Interpolate=off  OutputAfterFinalValue=Holding final value
  pitchrate_error : Outport
  pitchrate : Outport  Port=2
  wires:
  From Workspace2/1 -> pitchrate_error/1
  From Workspace1/1 -> pitchrate/1

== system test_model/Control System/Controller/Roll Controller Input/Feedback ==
  roll_error_model : Inport
  roll_angle_model : Inport  Port=2
  roll_error : Outport
  roll_angle : Outport  Port=2
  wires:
  roll_error_model/1 -> roll_error/1
  roll_angle_model/1 -> roll_angle/1
